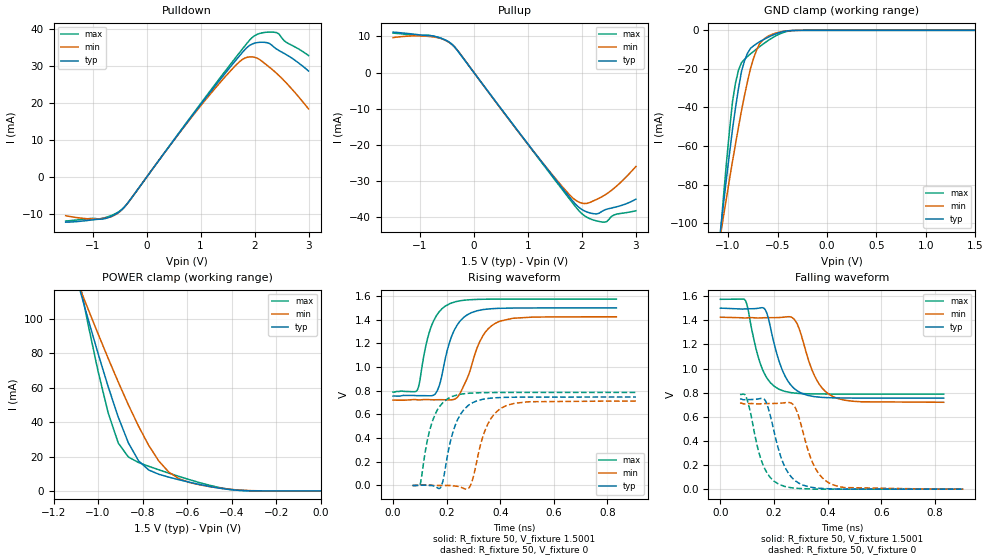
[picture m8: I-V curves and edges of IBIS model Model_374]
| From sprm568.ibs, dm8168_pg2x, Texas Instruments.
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| Model based on original model for BSHTLTCSCDDVGPBFZ
|   Sub model FASTEST_8MA_5PER_P_1P5
[model]   Model_374
|[Description]  [1.5V-3-STATE-X-FASTEST:8MA, IND, 5%]
|   Fastest slew rate (SR[1:0] = "00"), 1.00 * RExt = 1.000 * Iout
|   (I[2:0] = "011"), 8mA nominal with Rext = 50R, ,Industrial
|   temperature range (-40C to 125C, 25C nominal),5% power supply
|   tolerance
|[Input Load]
|[Output Drive] FASTEST:8MA
|Voltage   1.5V
|Mode   3-STATE
Model_type   3-state
Polarity   Non-Inverting
Enable   Active-Low
Cref =  15.0000pF
Rref =  100.0000M
Vref =  0V
Vmeas =  0.75005
C_comp   1.5249p   1.4275p   1.6205p
[Model Spec]
[Temperature Range]   25   125   -40
[Voltage Range]   1.5   1.425   1.575
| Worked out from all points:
|   slope of the pulldown table from 0 to 0.225 V, typ, clamps not added: 50.1 ohm
|   slope of the pullup table from 0 to 0.225 V, typ, clamps not added: 50.1 ohm
|   GND clamp passes 1 mA (typ) near -0.47 V on its own axis
|   POWER clamp passes 1 mA (typ) near -0.42 V on its own axis
|   rising waveform, R_fixture 50, V_fixture 1.5001: 20-80 % time 58.3ps typ, 73.3ps min, 53.6ps max; typ from 0.756 V to 1.5 V
|   rising waveform, R_fixture 50, V_fixture 0: 20-80 % time 55.5ps typ, 59.9ps min, 51.5ps max; typ from 0 V to 0.747 V
|   falling waveform, R_fixture 50, V_fixture 1.5001: 20-80 % time 63.9ps typ, 71.1ps min, 58.2ps max; typ from 1.5 V to 0.755 V
|   falling waveform, R_fixture 50, V_fixture 0: 20-80 % time 61.7ps typ, 66.4ps min, 55.6ps max; typ from 0.747 V to 0 V
[POWER_clamp]
-1.5V     321.7mA    260.6mA    415.9mA
-1.076V   114.2mA    115.8mA    116.9mA
-1.061V   107.2mA    110.9mA    107.1mA
-954.6mV  60.59mA    77.06mA    45.35mA
-909.2mV  42.85mA    63.21mA    27.81mA
-863.7mV  27.9mA     49.99mA    19.69mA
-818.2mV  17.49mA    37.63mA    16.52mA
-772.8mV  12.19mA    26.53mA    14.33mA
-681.9mV  7.985mA    10.89mA    10.33mA
-590.9mV  5.094mA    4.955mA    6.6mA
-363.7mV  298.5uA    465.2uA    297.6uA
0V        1.518nA    24.08nA    367.8pA
[Pulldown]
-1.5V     -12.15mA   -10.4mA    -11.83mA
-863.7mV  -11.34mA   -11.22mA   -11.25mA
-500mV    -9.267mA   -9.352mA   -9.148mA
-318.2mV  -6.354mA   -6.371mA   -6.385mA
1.046V    20.42mA    20.05mA    20.72mA
1.591V    30.47mA    29.26mA    31.18mA
1.818V    34.39mA    32.13mA    35.4mA
1.955V    35.92mA    32.45mA    37.67mA
2.091V    36.38mA    31.76mA    38.77mA
2.273V    36.08mA    29.69mA    39.15mA
2.364V    35.03mA    28.59mA    39.11mA
3V        28.64mA    18.41mA    32.82mA
[Pullup]
-1.5V     11.21mA    9.69mA     10.94mA
-818.2mV  10.23mA    9.978mA    10.29mA
-590.9mV  9.401mA    9.328mA    9.374mA
-409.1mV  7.828mA    7.781mA    7.859mA
1.227V    -24.14mA   -24.11mA   -24.35mA
1.727V    -33.63mA   -33.09mA   -34.13mA
1.909V    -36.81mA   -35.55mA   -37.6mA
2.046V    -38.25mA   -36.2mA    -39.57mA
2.227V    -39.04mA   -35.36mA   -40.83mA
2.409V    -38.05mA   -33.98mA   -41.36mA
2.591V    -37.29mA   -32.03mA   -39.38mA
3V        -34.98mA   -25.95mA   -38.2mA
[GND_clamp]
-1.5V     -310.1mA   -250.5mA   -402.5mA
-1.076V   -103.6mA   -106.2mA   -105.2mA
-1.046V   -89.81mA   -96.36mA   -86.02mA
-954.6mV  -51.22mA   -67.87mA   -36.88mA
-924.3mV  -40.08mA   -58.86mA   -27.29mA
-863.7mV  -21.24mA   -41.56mA   -16.73mA
-833.4mV  -15.8mA    -33.75mA   -15.03mA
-772.8mV  -9.345mA   -19.75mA   -12.19mA
-712.2mV  -6.928mA   -10.35mA   -9.704mA
-621.3mV  -4.261mA   -3.896mA   -6.225mA
-409.1mV  -337.1uA   -289.1uA   -618.9uA
1.5V      1.518nA    257.2nA    299pA
[Ramp]
dV/dt_f   0.600016/0.10061207n   0.567752/0.11362969n   0.630472/91.451266p
dV/dt_r  0.6179528/90.31641p   0.5951272/98.680182p  0.6425552/82.389602p
R_load = 50
[Rising Waveform]
R_fixture = 50
V_fixture = 1.5001
V_fixture_min = 1.425
V_fixture_max = 1.575
0s        755.9mV    721.1mV    789.3mV
90.52ps   759.1mV    724.1mV    806.9mV
129.2ps   758.1mV    725.9mV    1.246V
156.9ps   771.8mV    724.2mV    1.414V
176.1ps   870.6mV    724.7mV    1.477V
213.5ps   1.227V     723.2mV    1.538V
276ps     1.441V     901.8mV    1.567V
323.1ps   1.481V     1.213V     1.573V
381.7ps   1.495V     1.37V      1.574V
833.3ps   1.5V       1.425V     1.575V
[Rising Waveform]
R_fixture = 50
V_fixture = 0
V_fixture_min = 0
V_fixture_max = 0
72.99ps   0V         0V         0V
100.1ps   2.49mV     2.669mV    0V
135.7ps   0V         4.025mV    456.5mV
177.2ps   -18.19mV   0V         676.6mV
222.1ps   439.6mV    0V         753.3mV
251.5ps   600.8mV    -13.44mV   770.3mV
288.4ps   688.5mV    -2.664mV   780.1mV
343.2ps   731.1mV    465.1mV    784.4mV
416.1ps   744.4mV    668.3mV    785.9mV
906.3ps   747.3mV    712.8mV    786.3mV
[Falling Waveform]
R_fixture = 50
V_fixture = 1.5001
V_fixture_min = 1.425
V_fixture_max = 1.575
0s        1.501V     1.426V     1.575V
92.97ps   1.495V     1.419V     1.566V
137.1ps   1.499V     1.419V     1.129V
162.2ps   1.501V     1.422V     968.2mV
179.1ps   1.417V     1.422V     904.8mV
219ps     1.061V     1.423V     828mV
275.6ps   834.6mV    1.409V     797.7mV
350.9ps   767.3mV    942.2mV    790mV
420.7ps   757.4mV    767mV      788.8mV
833.3ps   755.2mV    720.6mV    788.5mV
[Falling Waveform]
R_fixture = 50
V_fixture = 0
V_fixture_min = 0
V_fixture_max = 0
72.99ps   747.4mV    713.5mV    785.8mV
96.91ps   742.5mV    707.7mV    760.3mV
143.7ps   749.3mV    707.2mV    304.7mV
168ps     733.4mV    709.8mV    159.2mV
219.2ps   312.7mV    712.2mV    39.28mV
245.4ps   164mV      717.9mV    20.12mV
276ps     75.5mV     688.5mV    9.219mV
351.2ps   11.84mV    186.4mV    0V
420.5ps   2.245mV    35.78mV    0V
906.3ps   0V         0V         0V
